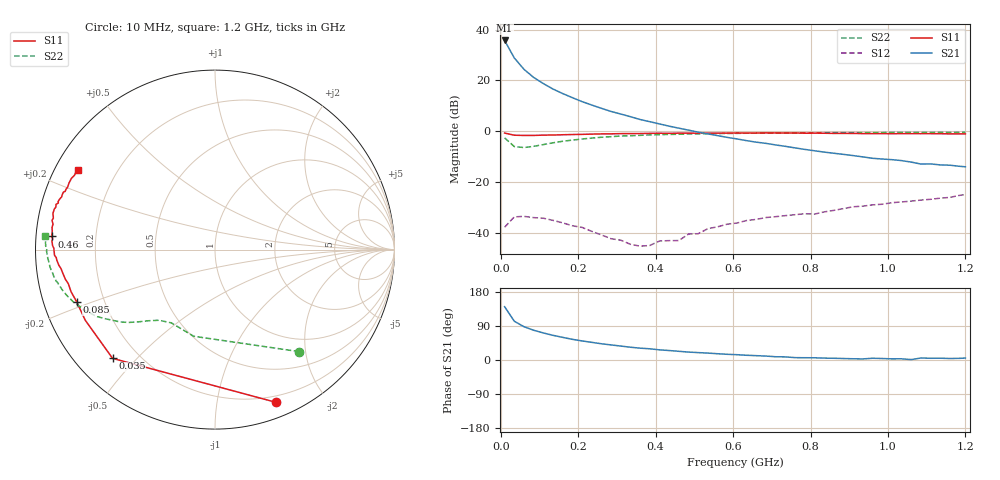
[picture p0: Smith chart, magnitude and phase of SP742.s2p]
!  POLYFET RF DEVICES
!  SP742, SQ742
!  S PARAMETERS
!  VDS=50V, IDQ=300mA
# MHZ S MA R 50
! Freq=Mhz Mag[s11] Ang[s11] Mag[s21] Ang[s21] Mag[s12] Ang[s12] Mag[s22] Ang[s22]
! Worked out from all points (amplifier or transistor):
!   49 points, 10 MHz to 1.2 GHz, reference 50 ohm
!   highest |S21| = 35.8 dB at 10 MHz (marker M1)
!   |S21| within 3 dB of that: start of sweep to 20.86 MHz
!   unconditionally stable (mu >= 1): 238.8 MHz to end of sweep
!   at 210 MHz: K = 0.75, MSG = 24.8 dB, |S12| = -38.0 dB
!   at 610 MHz: K = 1.49, MAG = 12.5 dB, |S12| = -36.3 dB
!   at 1.2 GHz: K = 1.60, MAG = 0.9 dB, |S12| = -25.0 dB
!   S11 on the Smith chart (normalised r, x): 10 MHz: 0.14, -1.47; 35 MHz: 0.11, -0.43; 85 MHz: 0.10, -0.18; 460 MHz: 0.05, +0.04; 1.2 GHz: 0.07, +0.27
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10  0.9173 -68.2  61.64 140.7  0.01273 49.3  0.7373 -50.5
35  0.8324 -133.3  27.83 102.4  0.02037 16.4  0.4972 -103.9
60  0.8231 -151.5  16.61 87.8  0.02084 3.2  0.4752 -120.8
85  0.8238 -159.3  11.5 78.5  0.01969 -3.3  0.5023 -128.4
110  0.8356 -163.8  8.686 71.4  0.01917 -8.7  0.5433 -133.1
135  0.839 -166.9  6.776 65.1  0.01736 -13.3  0.5896 -136.9
160  0.85 -168.8  5.518 59.7  0.01553 -15.8  0.6319 -140.0
185  0.8584 -171.3  4.583 54.6  0.01359 -18.3  0.6667 -142.9
210  0.8647 -173.0  3.829 50.3  0.01263 -16.9  0.6999 -145.9
235  0.8742 -174.2  3.28 46.6  0.01056 -13.6  0.7298 -148.3
260  0.883 -176.1  2.824 42.9  0.00897 -6.6  0.7581 -150.6
285  0.8857 -177.1  2.447 39.8  0.00755 -4.7  0.7785 -152.9
335  0.8965 -179.4  1.929 33.7  0.00586 16.7  0.8125 -156.5
360  0.8981 179.5  1.698 31.2  0.00538 28.7  0.8275 -158.4
410  0.9097 176.9  1.389 26.8  0.00681 52.8  0.8525 -161.4
460  0.913 175.4  1.145 22.9  0.00694 69.4  0.8688 -163.6
485  0.9123 174.4  1.048 20.9  0.00934 80.8  0.88 -165.2
610  0.9224 169.8  0.7029 14.0  0.01538 92.4  0.9052 -169.7
685  0.9253 167.4  0.5744 10.3  0.01977 91.2  0.9166 -172.4
810  0.914 163.0  0.4108 5.9  0.02307 99.4  0.9292 -176.1
1010  0.8918 156.9  0.2742 3.0  0.03876 101.5  0.9439 178.8
1200  0.8845 149.8  0.1981 5.1  0.05612 96.9  0.9487 175.4
